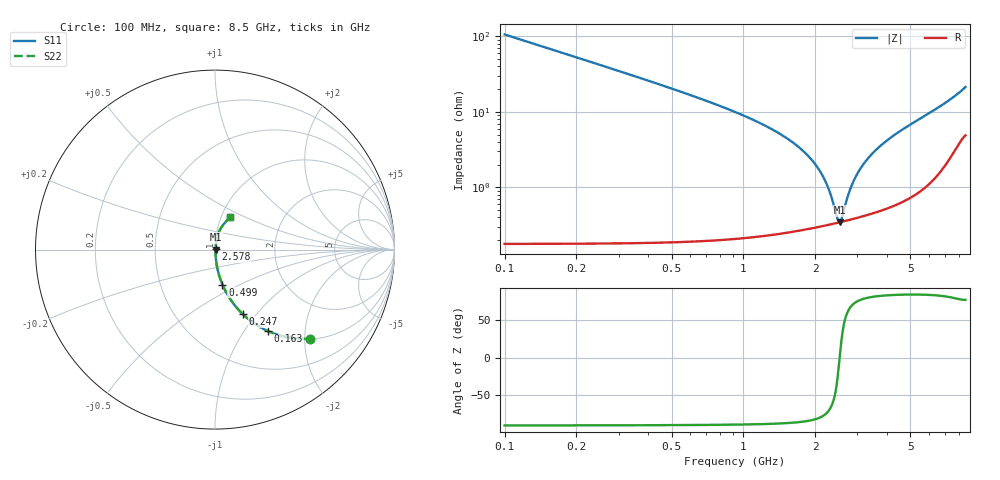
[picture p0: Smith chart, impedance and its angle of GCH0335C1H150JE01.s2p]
!Murata Part Number: GCH0335C1H150JE01
!These Parameters are Measured in Series Mode Connection
!Data Generated on Mar 13, 2026
!  o--ll--o
!Port1  Port2
!  o------o
!Operation Temp=25[degC], DC Bias Voltage=0[V]
!Freq. Start=100[MHz] Stop=9[GHz] 401[Steps]
# Hz S RI R 50
!Freq.(Hz) S11(Real) S11(Imag) S21(Real) S21(Imag) S12(Real) S12(Imag) S22(Real) S22(Imag)
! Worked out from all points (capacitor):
!   401 points, 100 MHz to 8.5 GHz, reference 50 ohm
!   read as one part in series: C = 15 pF near 142 MHz
!   lowest |Z| = 347 mohm at 2.536 GHz (marker M1)
!   series resonance near 2.529 GHz, so ESL is about 260 pH
!   S11 on the Smith chart (normalised r, x): 100 MHz: 1.00, -2.12; 163 MHz: 1.00, -1.30; 247 MHz: 1.00, -0.85; 499 MHz: 1.00, -0.41; 2.578 GHz: 1.01, +0.00; 8.5 GHz: 1.10, +0.42
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1e8  0.5288 -0.4983  0.4712 0.4983  0.4712 0.4983  0.5288 -0.4983
1.63e8  0.2964 -0.4553  0.7036 0.4553  0.7036 0.4553  0.2964 -0.4553
2.47e8  0.1543 -0.3592  0.8457 0.3592  0.8457 0.3592  0.1543 -0.3592
3.52e8  0.0818 -0.2709  0.9182 0.2709  0.9182 0.2709  0.0818 -0.2709
4.99e8  0.0417 -0.1955  0.9583 0.1955  0.9583 0.1955  0.0417 -0.1955
8.35e8  0.0146 -0.1114  0.9854 0.1114  0.9854 0.1114  0.0146 -0.1114
1.507e9  0.00454 -0.0452  0.9955 0.0452  0.9955 0.0452  0.00454 -0.0452
1.843e9  0.00351 -0.0269  0.9965 0.0269  0.9965 0.0269  0.00351 -0.0269
2.095e9  0.00327 -0.0159  0.9967 0.0159  0.9967 0.0159  0.00327 -0.0159
2.284e9  0.00327 -0.00857  0.9967 0.00857  0.9967 0.00857  0.00327 -0.00857
2.473e9  0.00339 -0.00188  0.9966 0.00188  0.9966 0.00188  0.00339 -0.00188
2.536e9  0.00345 0.000244  0.9966 -0.000244  0.9966 -0.000244  0.00345 0.000244
2.578e9  0.00349 0.00163  0.9965 -0.00163  0.9965 -0.00163  0.00349 0.00163
2.746e9  0.00371 0.00698  0.9963 -0.00698  0.9963 -0.00698  0.00371 0.00698
2.914e9  0.00399 0.0121  0.996 -0.0121  0.996 -0.0121  0.00399 0.0121
3.145e9  0.00445 0.0187  0.9955 -0.0187  0.9955 -0.0187  0.00445 0.0187
3.439e9  0.00517 0.0267  0.9948 -0.0267  0.9948 -0.0267  0.00517 0.0267
3.817e9  0.0063 0.0366  0.9937 -0.0366  0.9937 -0.0366  0.0063 0.0366
4.3e9  0.00812 0.0487  0.9919 -0.0487  0.9919 -0.0487  0.00812 0.0487
5.707e9  0.0169 0.0848  0.9831 -0.0848  0.9831 -0.0848  0.0169 0.0848
7.114e9  0.0374 0.1269  0.9626 -0.1269  0.9626 -0.1269  0.0374 0.1269
8.5e9  0.0827 0.182  0.9173 -0.182  0.9173 -0.182  0.0827 0.182
